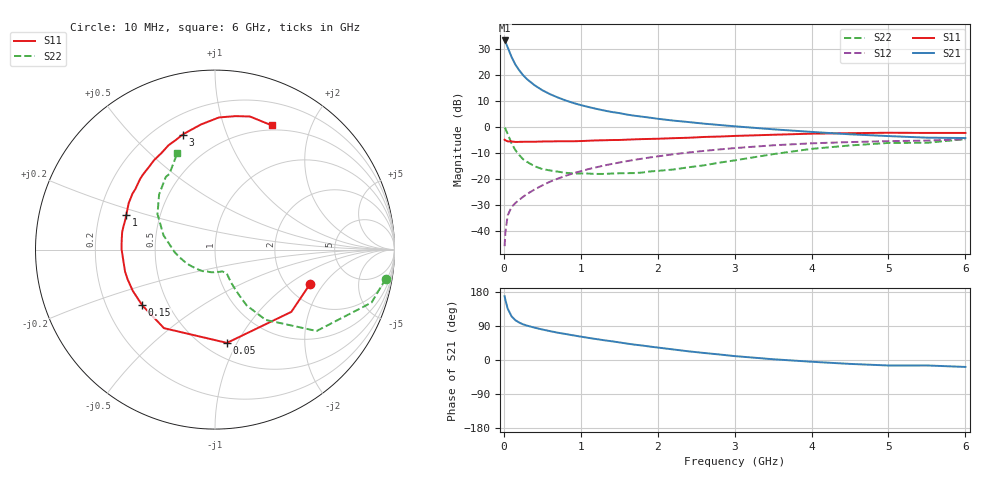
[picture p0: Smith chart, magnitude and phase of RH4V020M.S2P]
! SIEMENS Small Signal Semiconductors
! BFR106
! Si NPN RF Bipolar Junction Transistor in SOT23
! VCE = 4 V  IC = 20 mA
! Common Emitter S-Parameters:  August  1996
# GHz  S  MA  R  50
!  f  S11  S21  S12  S22
! GHz  MAG  ANG  MAG  ANG  MAG  ANG  MAG  ANG
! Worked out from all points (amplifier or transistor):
!   36 points, 10 MHz to 6 GHz, reference 50 ohm
!   highest |S21| = 33.1 dB at 10 MHz (marker M1)
!   |S21| within 3 dB of that: start of sweep to 54.82 MHz
!   unconditionally stable (mu >= 1): 366.7 MHz to 2.172 GHz
!   at 250 MHz: K = 0.89, MSG = 23.3 dB, |S12| = -26.9 dB
!   at 1.4 GHz: K = 1.07, MAG = 8.4 dB, |S12| = -14.3 dB
!   at 6 GHz: K = 1.00, MSG = 0.2 dB, |S12| = -4.8 dB
!   S11 on the Smith chart (normalised r, x): 10 MHz: 2.63, -1.49; 50 MHz: 0.64, -0.91; 150 MHz: 0.36, -0.30; 1 GHz: 0.32, +0.17; 3 GHz: 0.31, +0.71; 6 GHz: 0.44, +1.46
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0.01  0.5627 -20.1  45.32 168.3  0.0051 84.1  0.965 -9.7
0.02  0.5488 -39.2  43 158.7  0.0094 76.2  0.9207 -18.7
0.05  0.524 -82.7  33.42 135.5  0.0199 61.2  0.7253 -38.7
0.1  0.5219 -123.0  21.87 115.5  0.0287 53.0  0.4829 -54.2
0.15  0.5106 -142.6  15.6 104.9  0.0344 53.2  0.3564 -60.5
0.2  0.5125 -153.4  12.11 98.8  0.0395 55.6  0.2861 -62.1
0.25  0.5142 -161.2  9.773 94.1  0.0452 57.8  0.2383 -63.2
0.3  0.5158 -166.4  8.22 90.8  0.0509 60.6  0.2123 -63.8
0.4  0.5151 -174.8  6.252 85.3  0.0626 63.5  0.1744 -63.9
0.5  0.5209 179.6  5.029 80.5  0.0748 65.0  0.1541 -63.7
0.6  0.5226 174.0  4.223 76.2  0.0881 65.8  0.145 -65.2
0.8  0.5261 165.9  3.208 68.7  0.1139 66.0  0.1307 -70.2
1  0.531 158.4  2.606 61.7  0.14 65.1  0.1271 -75.8
1.1  0.5385 154.7  2.392 58.4  0.1538 64.4  0.1261 -80.7
1.3  0.5503 148.5  2.054 52.2  0.1797 62.5  0.1243 -88.6
1.6  0.5646 139.7  1.712 43.4  0.2186 59.2  0.1285 -103.8
2.2  0.6032 124.2  1.314 27.9  0.2956 51.4  0.1508 -136.5
3  0.6661 105.7  1.02 10.3  0.3891 39.5  0.2261 -176.7
3.5  0.7016 96.4  0.893 2.0  0.4403 31.9  0.2977 164.5
4.5  0.7523 81.3  0.716 -10.3  0.5077 16.3  0.4375 135.4
5.5  0.7604 69.3  0.617 -14.4  0.5431 6.0  0.492 121.1
6  0.761 65.5  0.607 -18.3  0.5752 -1.5  0.5786 111.2
